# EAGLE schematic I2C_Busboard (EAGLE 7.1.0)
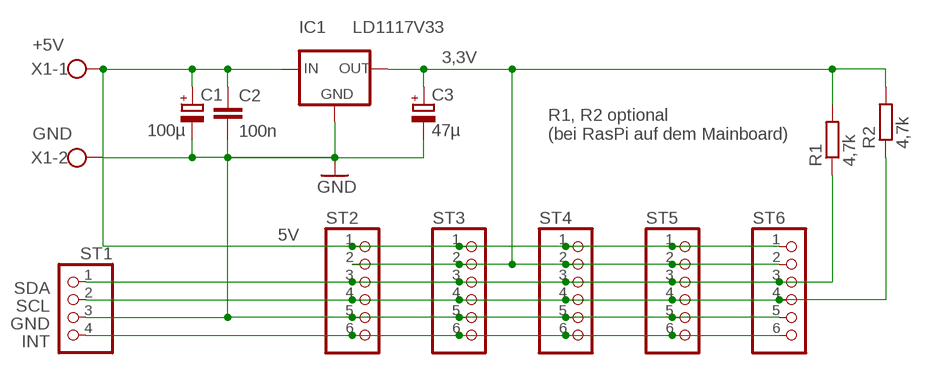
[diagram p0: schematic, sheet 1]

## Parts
C1  100µ  CPOL-EUE2-5  [E2-5]
C2  100n  C-EU025-025X050  [C025-025X050]
C3  47µ  CPOL-EUE2-5  [E2-5]
IC1  LD1117V33  78XXS  [78XXS]
R1  4,7k  R-EU_0204/7  [0204/7]
R2  4,7k  R-EU_0204/7  [0204/7]
ST1  PINHD-1X4  [1X04]
ST2  PINHD-1X6  [1X06]
ST3  PINHD-1X6  [1X06]
ST4  PINHD-1X6  [1X06]
ST5  PINHD-1X6  [1X06]
ST6  PINHD-1X6  [1X06]
X1  W237-102  [W237-102]

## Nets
GND: C1.- C2.2 C3.- IC1.GND ST1.3 ST2.5 ST3.5 ST4.5 ST5.5 ST6.5 X1.2
N$1: R2.1 ST1.2 ST2.4 ST3.4 ST4.4 ST5.4 ST6.4
N$4: ST1.4 ST2.6 ST3.6 ST4.6 ST5.6 ST6.6
N$7: R1.1 ST1.1 ST2.3 ST3.3 ST4.3 ST5.3 ST6.3
VCC: C3.+ IC1.OUT R1.2 R2.2 ST2.2 ST3.2 ST4.2 ST5.2 ST6.2
VCC1: C1.+ C2.1 IC1.IN ST2.1 ST3.1 ST4.1 ST5.1 ST6.1 X1.1

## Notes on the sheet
- +5V | 3,3V
- GND
- R1, R2 optional
  (bei RasPi auf dem Mainboard)
- 5V
- SDA
- SCL
- GND
- INT

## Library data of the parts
C1 C3 = rcl:CPOL-EU: POLARIZED CAPACITOR, European symbol
C2 = rcl:C-EU: CAPACITOR, European symbol
IC1 = v-reg:78XXS: VOLTAGE REGULATOR
R1 R2 = rcl:R-EU_: RESISTOR, European symbol
ST1 = pinhead:PINHD-1X4: PIN HEADER
ST2-ST6 = pinhead:PINHD-1X6: PIN HEADER
X1 = con-wago-500:W237-102: WAGO SCREW CLAMP; MPN: 237-102; OC_FARNELL: unknown; OC_NEWARK: 70K9898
